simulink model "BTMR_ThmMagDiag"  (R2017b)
settings: Solver=FixedStepDiscrete  StartTime=0.0  StopTime=10  FixedStep=0.1  RelTol=1e-3  EnableMultiTasking=on
undefined symbols (not defined in the file or in its folder): bin2dec, BTMR_cntHtgCoolDiag_CW, BTMR_tAChrgHtgDiag_C, BTMR_tCoolDiag_CUR, BTMR_tDChrgHtgDiag_C, BTMR_tEnvTCool_CUR, BTMR_tHeatDiag_CUR, BTMR_tiThmCoolDebDiag_C, BTMR_tiThmCoolDiag_C, BTMR_tiThmCoolEndDiag_C, BTMR_tiThmHtgDebDiag_C, BTMR_tiThmHtgDiag_C, BTMR_tiThmHtgEndDiag_C, BTMR_tLowClntDiag_CUR, BTMR_tThmCoolLowLimt_C, enmThmDiagFlg
libraries: simulink x22

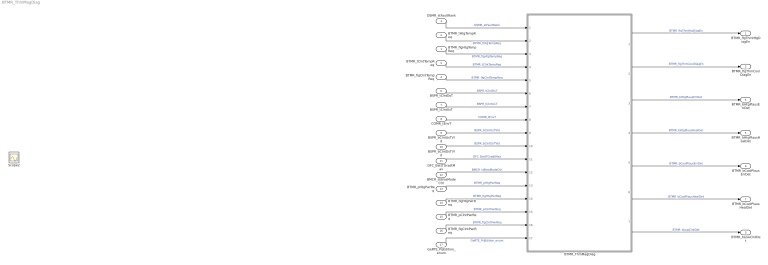
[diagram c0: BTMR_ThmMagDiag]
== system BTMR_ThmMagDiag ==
  BTMR_flgHtgTempReq : Inport
  BTMR_tHtgTempReq : Inport  Port=2
  DSMR_stFaultRank : Inport  Port=3
  BTMR_flgClntTempReq : Inport  Port=4
  BTMR_tClntTempReq : Inport  Port=5
  BSPR_tClntDsT : Inport  Port=6
  BSPR_tClntUsT : Inport  Port=7
  COMR_tEnvT : Inport  Port=8
  BSPR_bClntUsTVld : Inport  Port=9
  BSPR_bClntDsTVld : Inport  Port=10
  DFC_BattTGradtMax : Inport  Port=11
  BMCR_stBmsModeCtrl : Inport  Port=12
  BTMR_pHtgPwrReq : Inport  Port=13
  BTMR_flgHtgPwrReq : Inport  Port=14
  BTMR_pClntPwrReq : Inport  Port=15
  BTMR_flgClntPwrReq : Inport  Port=16
  GeRTE_PrjEdition_enum : Inport  Port=17
  BTMR_ThmMagDiag : Subsystem
  BTMR_flgThmHtgDiagEn : Outport
  BTMR_flgThmCoolDiagEn : Outport  Port=2
  BTMR_bLowClntDet : Outport  Port=3
  BTMR_bHtgPlausErrDet : Outport  Port=4
  BTMR_bHtgPlausHealDet : Outport  Port=5
  BTMR_bCoolPlausErrDet : Outport  Port=6
  BTMR_bCoolPlausHealDet : Outport  Port=7
  Scope2 : Scope
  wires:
  BTMR_tHtgTempReq/1 -> BTMR_ThmMagDiag/2(BTMR_tHtgTempReq)  "BTMR_tHtgTempReq"
  BTMR_flgHtgTempReq/1 -> BTMR_ThmMagDiag/3(BTMR_flgHtgTempReq)  "BTMR_flgHtgTempReq"
  BTMR_ThmMagDiag/1(BTMR_flgThmHtgDiagEn) -> BTMR_flgThmHtgDiagEn/1  "BTMR_flgThmHtgDiagEn"
  BTMR_ThmMagDiag/2(BTMR_flgThmCoolDiagEn) -> BTMR_flgThmCoolDiagEn/1  "BTMR_flgThmCoolDiagEn"
  BTMR_ThmMagDiag/4(BTMR_bHtgPlausHealDet) -> BTMR_bHtgPlausHealDet/1  "BTMR_bHtgPlausHealDet"
  BTMR_ThmMagDiag/3(BTMR_bHtgPlausErrDet) -> BTMR_bHtgPlausErrDet/1  "BTMR_bHtgPlausErrDet"
  BTMR_ThmMagDiag/5(BTMR_bCoolPlausErrDet) -> BTMR_bCoolPlausErrDet/1  "BTMR_bCoolPlausErrDet"
  BTMR_ThmMagDiag/6(BTMR_bCoolPlausHealDet) -> BTMR_bCoolPlausHealDet/1  "BTMR_bCoolPlausHealDet"
  BTMR_ThmMagDiag/7(BTMR_bLowClntDet) -> BTMR_bLowClntDet/1  "BTMR_bLowClntDet"
  DSMR_stFaultRank/1 -> BTMR_ThmMagDiag/1(DSMR_stFaultRank)  "DSMR_stFaultRank"
  BTMR_tClntTempReq/1 -> BTMR_ThmMagDiag/4(BTMR_tClntTempReq)  "BTMR_tClntTempReq"
  BTMR_flgClntTempReq/1 -> BTMR_ThmMagDiag/5(BTMR_flgClntTempReq)  "BTMR_flgClntTempReq"
  BSPR_tClntDsT/1 -> BTMR_ThmMagDiag/6(BSPR_tClntDsT)  "BSPR_tClntDsT"
  BSPR_tClntUsT/1 -> BTMR_ThmMagDiag/7(BSPR_tClntUsT)  "BSPR_tClntUsT"
  COMR_tEnvT/1 -> BTMR_ThmMagDiag/8(COMR_tEnvT)  "COMR_tEnvT"
  BSPR_bClntUsTVld/1 -> BTMR_ThmMagDiag/9(BSPR_bClntUsTVld)  "BSPR_bClntUsTVld"
  BSPR_bClntDsTVld/1 -> BTMR_ThmMagDiag/10(BSPR_bClntDsTVld)  "BSPR_bClntDsTVld"
  DFC_BattTGradtMax/1 -> BTMR_ThmMagDiag/11(DFC_BattTGradtMax)  "DFC_BattTGradtMax"
  BMCR_stBmsModeCtrl/1 -> BTMR_ThmMagDiag/12(BMCR_stBmsModeCtrl)  "BMCR_stBmsModeCtrl"
  BTMR_pHtgPwrReq/1 -> BTMR_ThmMagDiag/13(BTMR_pHtgPwrReq)  "BTMR_pHtgPwrReq"
  BTMR_flgHtgPwrReq/1 -> BTMR_ThmMagDiag/14(BTMR_flgHtgPwrReq)  "BTMR_flgHtgPwrReq"
  BTMR_flgClntPwrReq/1 -> BTMR_ThmMagDiag/16(BTMR_flgClntPwrReq)  "BTMR_flgClntPwrReq"
  BTMR_pClntPwrReq/1 -> BTMR_ThmMagDiag/15(BTMR_pClntPwrReq)  "BTMR_pClntPwrReq"
  GeRTE_PrjEdition_enum/1 -> BTMR_ThmMagDiag/17(GeRTE_PrjEdition_enum)  "GeRTE_PrjEdition_enum"

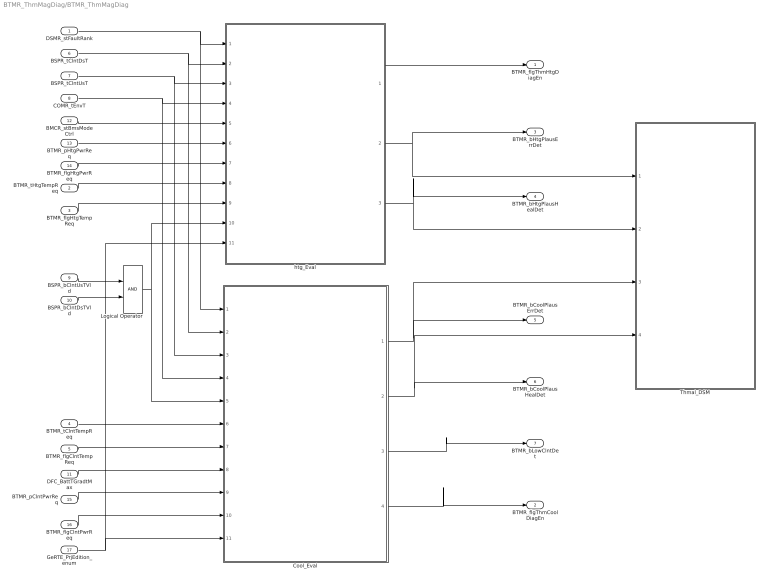
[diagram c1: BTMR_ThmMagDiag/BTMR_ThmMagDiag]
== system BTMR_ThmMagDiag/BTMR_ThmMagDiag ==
  DSMR_stFaultRank : Inport
  BTMR_tHtgTempReq : Inport  Port=2
  BTMR_flgHtgTempReq : Inport  Port=3
  BTMR_tClntTempReq : Inport  Port=4
  BTMR_flgClntTempReq : Inport  Port=5
  BSPR_tClntDsT : Inport  Port=6
  BSPR_tClntUsT : Inport  Port=7
  COMR_tEnvT : Inport  Port=8
  BSPR_bClntUsTVld : Inport  Port=9
  BSPR_bClntDsTVld : Inport  Port=10
  DFC_BattTGradtMax : Inport  Port=11  OutDataTypeStr=uint8
  BMCR_stBmsModeCtrl : Inport  Port=12
  BTMR_pHtgPwrReq : Inport  Port=13
  BTMR_flgHtgPwrReq : Inport  Port=14
  BTMR_pClntPwrReq : Inport  Port=15
  BTMR_flgClntPwrReq : Inport  Port=16
  GeRTE_PrjEdition_enum : Inport  Port=17
  Cool_Eval : Subsystem  TreatAsAtomicUnit=on
  Logical Operator : Logic  AllPortsSameDT=off  OutDataTypeStr=boolean
  Thmal_DSM : Subsystem
  htg_Eval : Subsystem  TreatAsAtomicUnit=on
  BTMR_flgThmHtgDiagEn : Outport
  BTMR_flgThmCoolDiagEn : Outport  Port=2
  BTMR_bHtgPlausErrDet : Outport  Port=3
  BTMR_bHtgPlausHealDet : Outport  Port=4
  BTMR_bCoolPlausErrDet : Outport  Port=5
  BTMR_bCoolPlausHealDet : Outport  Port=6
  BTMR_bLowClntDet : Outport  Port=7
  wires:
  DSMR_stFaultRank/1 -> Cool_Eval/1(DSMR_stFaultRank), htg_Eval/1(DSMR_stFaultRank)
  BSPR_tClntDsT/1 -> Cool_Eval/2(BSPR_tClntDsT), htg_Eval/2(BSPR_tClntDsT)
  BSPR_tClntUsT/1 -> Cool_Eval/3(BSPR_tClntUsT), htg_Eval/3(BSPR_tClntUsT)
  COMR_tEnvT/1 -> Cool_Eval/4(COMR_tEnvT), htg_Eval/4(COMR_tEnvT)
  htg_Eval/1(BTMR_flgThmHtgDiagEn) -> BTMR_flgThmHtgDiagEn/1
  BTMR_flgClntTempReq/1 -> Cool_Eval/7(BTMR_flgClntTempReq)
  BTMR_tClntTempReq/1 -> Cool_Eval/6(BTMR_tClntTempReq)
  BSPR_bClntUsTVld/1 -> Logical Operator/1
  BSPR_bClntDsTVld/1 -> Logical Operator/2
  Logical Operator/1 -> htg_Eval/10(BSPR_bClntTVld), Cool_Eval/5(BSPR_bClntTVld)
  Cool_Eval/3(BTMR_bLowClntDet) -> BTMR_bLowClntDet/1
  DFC_BattTGradtMax/1 -> Cool_Eval/8(DFC_BattTGradtMax)
  htg_Eval/2(BTMR_bHtgPlausErrDet) -> BTMR_bHtgPlausErrDet/1, Thmal_DSM/1(BTMR_bHtgPlausErrDet)
  htg_Eval/3(BTMR_bHtgPlausHealDet) -> BTMR_bHtgPlausHealDet/1, Thmal_DSM/2(BTMR_bHtgPlausHealDet)
  Cool_Eval/1(BTMR_bCoolPlausErrDet) -> Thmal_DSM/3(BTMR_bCoolPlausErrDet), BTMR_bCoolPlausErrDet/1
  Cool_Eval/2(BTMR_bCoolPlausHealDet) -> Thmal_DSM/4(BTMR_bCoolPlausHealDet), BTMR_bCoolPlausHealDet/1
  Cool_Eval/4(BTMR_flgThmCoolDiagEn) -> BTMR_flgThmCoolDiagEn/1
  BMCR_stBmsModeCtrl/1 -> htg_Eval/5(BMCR_stBmsModeCtrl)
  BTMR_pClntPwrReq/1 -> Cool_Eval/9(BTMR_pClntPwrReq)
  BTMR_flgClntPwrReq/1 -> Cool_Eval/10(BTMR_flgClntPwrReq)
  BTMR_pHtgPwrReq/1 -> htg_Eval/6(BTMR_pHtgPwrReq)
  BTMR_flgHtgPwrReq/1 -> htg_Eval/7(BTMR_flgHtgPwrReq)
  BTMR_flgHtgTempReq/1 -> htg_Eval/9(BTMR_flgHtgTempReq)
  BTMR_tHtgTempReq/1 -> htg_Eval/8(BTMR_tHtgTempReq)
  GeRTE_PrjEdition_enum/1 -> htg_Eval/11(GeRTE_PrjEdition_enum), Cool_Eval/11(GeRTE_PrjEdition_enum)

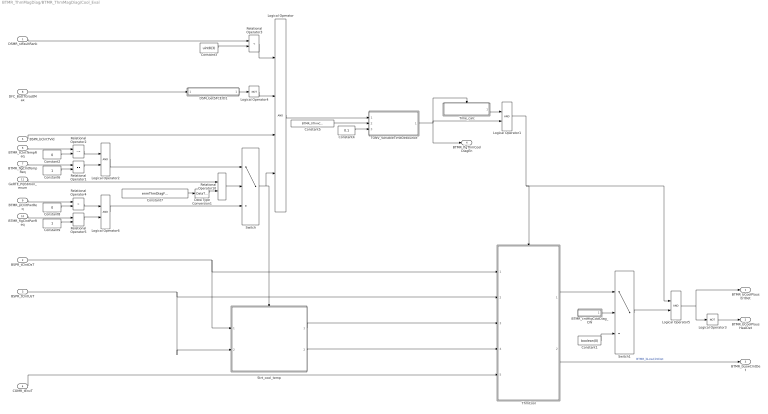
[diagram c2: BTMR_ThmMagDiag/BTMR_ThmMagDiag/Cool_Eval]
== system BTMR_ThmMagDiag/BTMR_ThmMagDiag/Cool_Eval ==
  DSMR_stFaultRank : Inport
  BSPR_tClntDsT : Inport  Port=2
  BSPR_tClntUsT : Inport  Port=3
  COMR_tEnvT : Inport  Port=4
  BSPR_bClntTVld : Inport  Port=5
  BTMR_tClntTempReq : Inport  Port=6
  BTMR_flgClntTempReq : Inport  Port=7
  DFC_BattTGradtMax : Inport  Port=8
  BTMR_pClntPwrReq : Inport  Port=9
  BTMR_flgClntPwrReq : Inport  Port=10
  GeRTE_PrjEdition_enum : Inport  Port=11
  BTMR_cntHtgCoolDiag_CW : Subsystem
  Constant1 : Constant  Value=boolean(0)
  Constant2 : Constant  Value=0  OutDataTypeStr=single
  Constant3 : Constant  Value=uint8(3)
  Constant4 : Constant  Value=0.1
  Constant5 : Constant  Value=BTMR_tiThmCoolDiag_C
  Constant6 : Constant  OutDataTypeStr=boolean
  Constant7 : Constant  Value=enmThmDiagFlg.TempReq  OutDataTypeStr=Enum: enmThmDiagFlg
  Constant8 : Constant  Value=0  OutDataTypeStr=single
  Constant9 : Constant  OutDataTypeStr=boolean
  DSM_GetSFCErD1 : Subsystem  TreatAsAtomicUnit=on  RTWFcnName=TONV_10msTimeDebounce  RTWFileName=SrvLib
  Data Type Conversion1 : DataTypeConversion  OutDataTypeStr=uint8
  Logical Operator : Logic  Inputs=4  AllPortsSameDT=off  OutDataTypeStr=boolean
  Logical Operator{1..2,5..6} (4 alike) : Logic  AllPortsSameDT=off  OutDataTypeStr=boolean
  Logical Operator3 : Logic  Operator=NOT  Inputs=1  AllPortsSameDT=off  OutDataTypeStr=boolean
  Logical Operator4 : Logic  Operator=NOT  Inputs=1  AllPortsSameDT=off  OutDataTypeStr=boolean
  Relational Operator1 : RelationalOperator  Operator===  OutDataTypeStr=boolean  RndMeth=Simplest
  Relational Operator10 : RelationalOperator  Operator===  OutDataTypeStr=boolean  RndMeth=Simplest
  Relational Operator2 : RelationalOperator  Operator=~=  OutDataTypeStr=boolean  RndMeth=Simplest
  Relational Operator3 : RelationalOperator  Operator=<  OutDataTypeStr=boolean  RndMeth=Simplest
  Relational Operator4 : RelationalOperator  Operator=>  OutDataTypeStr=boolean  RndMeth=Simplest
  Relational Operator5 : RelationalOperator  Operator===  OutDataTypeStr=boolean  RndMeth=Simplest
  Strt_cool_temp : Subsystem  TreatAsAtomicUnit=on
  Switch : Switch  Criteria=u2 > Threshold
  Switch1 : Switch  Criteria=u2 > Threshold
  TONV_VariableTimeDebounce : Subsystem  TreatAsAtomicUnit=on  RTWFcnName=TONV_VariableTimeDebounce  RTWFileName=SrvLib
  ThmCool : Subsystem  TreatAsAtomicUnit=on
  Time_calc : Subsystem  TreatAsAtomicUnit=on
  BTMR_bCoolPlausErrDet : Outport
  BTMR_bCoolPlausHealDet : Outport  Port=2
  BTMR_bLowClntDet : Outport  Port=3
  BTMR_flgThmCoolDiagEn : Outport  Port=4
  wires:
  Constant2/1 -> Relational Operator2/2
  Constant3/1 -> Relational Operator3/2
  Constant4/1 -> TONV_VariableTimeDebounce/3(dT)
  Constant5/1 -> TONV_VariableTimeDebounce/2(T)
  Relational Operator2/1 -> Logical Operator2/1
  Relational Operator3/1 -> Logical Operator/1
  BSPR_tClntDsT/1 -> ThmCool/1(BSPR_tClntDsT), Strt_cool_temp/1(BSPR_tClntDsT)
  BSPR_tClntUsT/1 -> ThmCool/2(BSPR_tClntUsT), Strt_cool_temp/2(BSPR_tClntUsT)
  DSMR_stFaultRank/1 -> Relational Operator3/1
  BTMR_tClntTempReq/1 -> Relational Operator2/1
  TONV_VariableTimeDebounce/1(y) -> Logical Operator1/2, BTMR_flgThmCoolDiagEn/1, Time_calc/Enable
  Time_calc/1(BTMR_flgThmCoolTimeEn) -> Logical Operator1/1
  Logical Operator1/1 -> Logical Operator5/1, ThmCool/Enable
  Constant1/1 -> Switch1/3
  ThmCool/1(BTMR_bCoolPlausErrDet) -> Switch1/1
  Logical Operator3/1 -> BTMR_bCoolPlausHealDet/1
  BTMR_cntHtgCoolDiag_CW/1(CW) -> Switch1/2
  Switch/1 -> Strt_cool_temp/Trigger, Logical Operator/4
  BSPR_bClntTVld/1 -> Logical Operator/3
  ThmCool/2(BTMR_bLowClntDet) -> BTMR_bLowClntDet/1  "BTMR_bLowClntDet"
  Strt_cool_temp/1(BSPR_tClntDsStrtCool) -> ThmCool/3(BSPR_tClntDsStrtCool)
  Strt_cool_temp/2(BSPR_tClntUsStrtCool) -> ThmCool/4(BSPR_tClntUsStrtCool)
  COMR_tEnvT/1 -> ThmCool/5(COMR_tEnvT)
  Logical Operator4/1 -> Logical Operator/2
  DFC_BattTGradtMax/1 -> DSM_GetSFCErD1/1(DFC)
  DSM_GetSFCErD1/1(y) -> Logical Operator4/1
  Logical Operator/1 -> TONV_VariableTimeDebounce/1(u)
  Switch1/1 -> Logical Operator5/2
  Logical Operator5/1 -> BTMR_bCoolPlausErrDet/1, Logical Operator3/1
  Constant6/1 -> Relational Operator1/2
  BTMR_flgClntTempReq/1 -> Relational Operator1/1
  Relational Operator1/1 -> Logical Operator2/2
  Relational Operator10/1 -> Switch/2
  Relational Operator4/1 -> Logical Operator6/1
  Constant8/1 -> Relational Operator4/2
  BTMR_pClntPwrReq/1 -> Relational Operator4/1
  Logical Operator2/1 -> Switch/1
  Logical Operator6/1 -> Switch/3
  BTMR_flgClntPwrReq/1 -> Relational Operator5/1
  Constant9/1 -> Relational Operator5/2
  Relational Operator5/1 -> Logical Operator6/2
  Data Type Conversion1/1 -> Relational Operator10/2
  GeRTE_PrjEdition_enum/1 -> Relational Operator10/1
  Constant7/1 -> Data Type Conversion1/1

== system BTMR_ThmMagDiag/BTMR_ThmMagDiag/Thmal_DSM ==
  BTMR_bHtgPlausErrDet : Inport
  BTMR_bHtgPlausHealDet : Inport  Port=2
  BTMR_bCoolPlausErrDet : Inport  Port=3
  BTMR_bCoolPlausHealDet : Inport  Port=4
  DSM_ReportCheck2 : Subsystem  TreatAsAtomicUnit=on  RTWFcnName=DSM_ReportCheck  RTWFileName=SrvLib
  DSM_ReportCheck3 : Subsystem  TreatAsAtomicUnit=on  RTWFcnName=DSM_ReportCheck  RTWFileName=SrvLib
  Data Store Read : DataStoreRead  DataStoreName=DFC_HtgPerfPlaus
  Data Store Read1 : DataStoreRead  DataStoreName=DFC_CoolPerfPlaus
  Data Store Write : DataStoreWrite  DataStoreName=DFC_HtgPerfPlaus
  Data Store Write1 : DataStoreWrite  DataStoreName=DFC_CoolPerfPlaus
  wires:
  DSM_ReportCheck2/1(Dfc_id) -> Data Store Write1/1
  Data Store Read1/1 -> DSM_ReportCheck2/1(Dfc_id_nv)
  Data Store Read/1 -> DSM_ReportCheck3/1(Dfc_id_nv)
  DSM_ReportCheck3/1(Dfc_id) -> Data Store Write/1
  BTMR_bHtgPlausErrDet/1 -> DSM_ReportCheck3/2(Err)
  BTMR_bHtgPlausHealDet/1 -> DSM_ReportCheck3/3(Heal)
  BTMR_bCoolPlausErrDet/1 -> DSM_ReportCheck2/2(Err)
  BTMR_bCoolPlausHealDet/1 -> DSM_ReportCheck2/3(Heal)

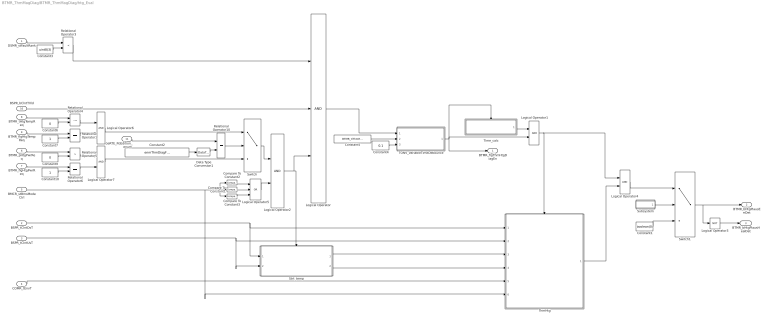
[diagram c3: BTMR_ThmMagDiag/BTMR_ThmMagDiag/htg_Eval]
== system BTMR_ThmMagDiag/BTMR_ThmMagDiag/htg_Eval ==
  DSMR_stFaultRank : Inport
  BSPR_tClntDsT : Inport  Port=2
  BSPR_tClntUsT : Inport  Port=3
  COMR_tEnvT : Inport  Port=4
  BMCR_stBmsModeCtrl : Inport  Port=5
  BTMR_pHtgPwrReq : Inport  Port=6
  BTMR_flgHtgPwrReq : Inport  Port=7
  BTMR_tHtgTempReq : Inport  Port=8
  BTMR_flgHtgTempReq : Inport  Port=9
  BSPR_bClntTVld : Inport  Port=10
  GeRTE_PrjEdition_enum : Inport  Port=11
  Compare To Constant1 : simulink/Logic and Bit Operations/Compare To Constant  relop===  const=5  OutDataTypeStr=boolean
  Compare To Constant2 : simulink/Logic and Bit Operations/Compare To Constant  relop===  const=6  OutDataTypeStr=boolean
  Compare To Constant3 : simulink/Logic and Bit Operations/Compare To Constant  relop===  const=11  OutDataTypeStr=boolean
  Constant1 : Constant  Value=boolean(0)
  Constant10 : Constant  OutDataTypeStr=boolean
  Constant2 : Constant  Value=enmThmDiagFlg.TempReq  OutDataTypeStr=Enum: enmThmDiagFlg
  Constant3 : Constant  Value=uint8(3)
  Constant4 : Constant  Value=0.1
  Constant5 : Constant  Value=BTMR_tiThmHtgDiag_C
  Constant6 : Constant  Value=0  OutDataTypeStr=single
  Constant7 : Constant  OutDataTypeStr=boolean
  Constant9 : Constant  Value=0  OutDataTypeStr=single
  Data Type Conversion1 : DataTypeConversion  OutDataTypeStr=uint8
  Logical Operator : Logic  Inputs=3  AllPortsSameDT=off  OutDataTypeStr=boolean
  Logical Operator{1..2,4,6..7} (5 alike) : Logic  AllPortsSameDT=off  OutDataTypeStr=boolean
  Logical Operator3 : Logic  Operator=NOT  Inputs=1  AllPortsSameDT=off  OutDataTypeStr=boolean
  Logical Operator5 : Logic  Operator=OR  Inputs=3  AllPortsSameDT=off  OutDataTypeStr=boolean
  Relational Operator1 : RelationalOperator  Operator===  OutDataTypeStr=boolean  RndMeth=Simplest
  Relational Operator10 : RelationalOperator  Operator===  OutDataTypeStr=boolean  RndMeth=Simplest
  Relational Operator3 : RelationalOperator  Operator=<  OutDataTypeStr=boolean  RndMeth=Simplest
  Relational Operator4 : RelationalOperator  Operator=~=  OutDataTypeStr=boolean  RndMeth=Simplest
  Relational Operator5 : RelationalOperator  Operator=>  OutDataTypeStr=boolean  RndMeth=Simplest
  Relational Operator6 : RelationalOperator  Operator===  OutDataTypeStr=boolean  RndMeth=Simplest
  Strt_temp : Subsystem  TreatAsAtomicUnit=on
  Subsystem : Subsystem
  Switch : Switch  Criteria=u2 > Threshold
  Switch1 : Switch  Criteria=u2 > Threshold
  TONV_VariableTimeDebounce : Subsystem  TreatAsAtomicUnit=on  RTWFcnName=TONV_VariableTimeDebounce  RTWFileName=SrvLib
  ThmHtg : Subsystem  TreatAsAtomicUnit=on
  Time_calc : Subsystem  TreatAsAtomicUnit=on
  BTMR_flgThmHtgDiagEn : Outport
  BTMR_bHtgPlausErrDet : Outport  Port=2
  BTMR_bHtgPlausHealDet : Outport  Port=3
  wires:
  DSMR_stFaultRank/1 -> Relational Operator3/1
  Constant3/1 -> Relational Operator3/2
  Logical Operator/1 -> TONV_VariableTimeDebounce/1(u)
  Constant4/1 -> TONV_VariableTimeDebounce/3(dT)
  Constant5/1 -> TONV_VariableTimeDebounce/2(T)
  TONV_VariableTimeDebounce/1(y) -> Logical Operator1/2, BTMR_flgThmHtgDiagEn/1, Time_calc/Enable
  COMR_tEnvT/1 -> ThmHtg/5(COMR_tEnvT)
  BSPR_tClntDsT/1 -> Strt_temp/1(BSPR_tClntDsT), ThmHtg/1(BSPR_tClntDsT)
  BSPR_tClntUsT/1 -> Strt_temp/2(BSPR_tClntUsT), ThmHtg/2(BSPR_tClntUsT)
  Strt_temp/2(BSPR_tClntUsStrtHtg) -> ThmHtg/4(BSPR_tClntUsStrtHtg)
  Strt_temp/1(BSPR_tClntDsStrtHtg) -> ThmHtg/3(BSPR_tClntDsStrtHtg)
  Relational Operator3/1 -> Logical Operator/1
  Time_calc/1(BTMR_flgThmHtgTimeEn) -> Logical Operator1/1
  Logical Operator1/1 -> ThmHtg/Enable, Logical Operator4/1
  Constant1/1 -> Switch1/3
  Switch1/1 -> Logical Operator3/1, BTMR_bHtgPlausErrDet/1
  Logical Operator3/1 -> BTMR_bHtgPlausHealDet/1
  Subsystem/1(CW) -> Switch1/2
  ThmHtg/1(BTMR_bHtgPlausErrDet) -> Logical Operator4/2
  Logical Operator4/1 -> Switch1/1
  BMCR_stBmsModeCtrl/1 -> ThmHtg/6(BMCR_stBmsModeCtrl), Compare To Constant3/1, Compare To Constant2/1, Compare To Constant1/1
  Logical Operator2/1 -> Strt_temp/Trigger, Logical Operator/3
  Compare To Constant2/1 -> Logical Operator5/1
  Compare To Constant1/1 -> Logical Operator5/2
  Logical Operator5/1 -> Logical Operator2/2
  Compare To Constant3/1 -> Logical Operator5/3
  Logical Operator7/1 -> Switch/3
  Relational Operator10/1 -> Switch/2
  Relational Operator4/1 -> Logical Operator6/1
  Relational Operator1/1 -> Logical Operator6/2
  Constant7/1 -> Relational Operator1/2
  Constant9/1 -> Relational Operator5/2
  BTMR_flgHtgTempReq/1 -> Relational Operator1/1
  Relational Operator5/1 -> Logical Operator7/1
  Logical Operator6/1 -> Switch/1
  Relational Operator6/1 -> Logical Operator7/2
  Constant10/1 -> Relational Operator6/2
  Constant6/1 -> Relational Operator4/2
  BTMR_tHtgTempReq/1 -> Relational Operator4/1
  BTMR_pHtgPwrReq/1 -> Relational Operator5/1
  BTMR_flgHtgPwrReq/1 -> Relational Operator6/1
  Switch/1 -> Logical Operator2/1
  BSPR_bClntTVld/1 -> Logical Operator/2
  Data Type Conversion1/1 -> Relational Operator10/2
  GeRTE_PrjEdition_enum/1 -> Relational Operator10/1
  Constant2/1 -> Data Type Conversion1/1

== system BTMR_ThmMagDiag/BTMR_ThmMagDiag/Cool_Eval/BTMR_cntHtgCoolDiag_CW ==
  Bitwise Operator : simulink/Logic and Bit Operations/Bitwise Operator  logicop=AND  UseBitMask=on  BitMask=bin2dec('00000010')  BitMaskRealWorld=Stored Integer
  Compare To Constant1 : simulink/Logic and Bit Operations/Compare To Constant  relop===  const=2  OutDataTypeStr=boolean
  Constant7 : Constant  Value=BTMR_cntHtgCoolDiag_CW
  CW : Outport
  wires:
  Compare To Constant1/1 -> CW/1
  Constant7/1 -> Bitwise Operator/1
  Bitwise Operator/1 -> Compare To Constant1/1

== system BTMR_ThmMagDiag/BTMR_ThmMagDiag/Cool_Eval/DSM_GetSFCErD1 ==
  DFC : Inport  OutDataTypeStr=uint8
  DFC_IsoChkLv1_1 : simulink/Logic and Bit Operations/Bitwise Operator  logicop=AND  UseBitMask=on  BitMask=bin2dec('00010000')  BitMaskRealWorld=Stored Integer
  DFC_IsoChkLv1_1_compare : simulink/Logic and Bit Operations/Compare To Constant  relop===  const=16  OutDataTypeStr=boolean
  y : Outport
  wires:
  DFC_IsoChkLv1_1/1 -> DFC_IsoChkLv1_1_compare/1
  DFC/1 -> DFC_IsoChkLv1_1/1
  DFC_IsoChkLv1_1_compare/1 -> y/1

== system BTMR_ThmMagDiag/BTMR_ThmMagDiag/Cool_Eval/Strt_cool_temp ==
  BSPR_tClntDsT : Inport
  BSPR_tClntUsT : Inport  Port=2
  Trigger : TriggerPort  VariantControl=Variant
  BSPR_tClntDsStrtCool : Outport
  BSPR_tClntUsStrtCool : Outport  Port=2
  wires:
  BSPR_tClntDsT/1 -> BSPR_tClntDsStrtCool/1  "BSPR_tClntDsStrtCool"
  BSPR_tClntUsT/1 -> BSPR_tClntUsStrtCool/1  "BSPR_tClntUsStrtCool"

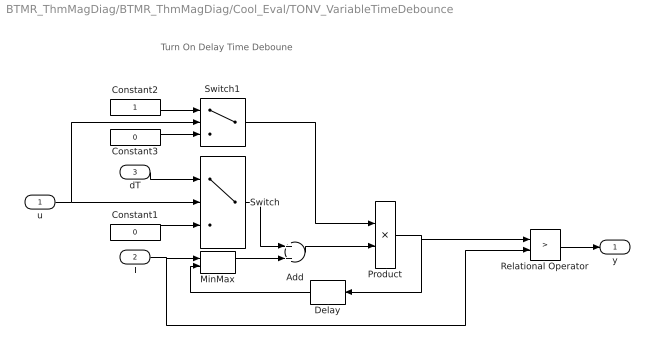
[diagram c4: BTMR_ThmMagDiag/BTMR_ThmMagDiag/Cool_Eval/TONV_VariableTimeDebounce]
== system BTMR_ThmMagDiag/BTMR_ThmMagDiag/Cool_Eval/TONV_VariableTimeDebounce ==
  note: Turn On Delay Time Deboune
  u : Inport
  T : Inport  Port=2
  dT : Inport  Port=3
  Add : Sum
  Constant1 : Constant  Value=0  OutDataTypeStr=single
  Constant2 : Constant  OutDataTypeStr=uint8
  Constant3 : Constant  Value=0  OutDataTypeStr=uint8
  Delay : Delay  DelayLength=1  InitialCondition=0
  MinMax : MinMax  Inputs=2
  Product : Product  OutMin=[0]  OutMax=[65535]  OutDataTypeStr=single
  Relational Operator : RelationalOperator  Operator=>  OutDataTypeStr=boolean  RndMeth=Simplest
  Switch : Switch  Criteria=u2 ~= 0
  Switch1 : Switch  Criteria=u2 ~= 0
  y : Outport
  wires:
  Switch1/1 -> Product/1
  Constant3/1 -> Switch1/3
  Constant2/1 -> Switch1/1
  u/1 -> Switch1/2, Switch/2
  dT/1 -> Switch/1
  Constant1/1 -> Switch/3
  Add/1 -> Product/2
  Product/1 -> Relational Operator/1, Delay/1
  Switch/1 -> Add/1
  Delay/1 -> MinMax/2
  Relational Operator/1 -> y/1
  T/1 -> MinMax/1, Relational Operator/2
  MinMax/1 -> Add/2

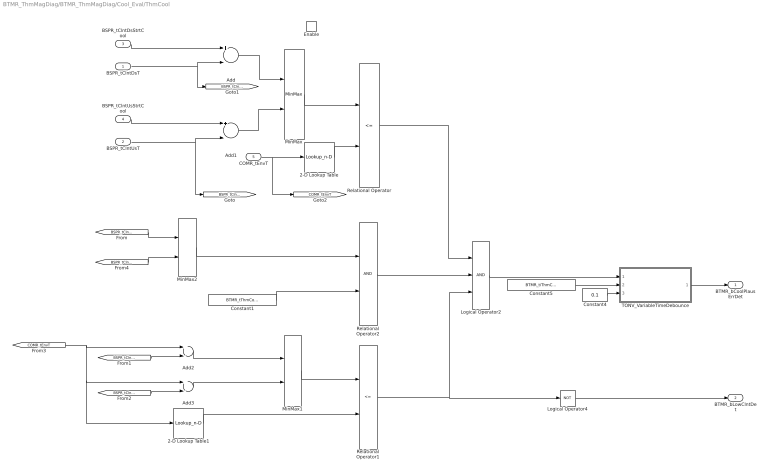
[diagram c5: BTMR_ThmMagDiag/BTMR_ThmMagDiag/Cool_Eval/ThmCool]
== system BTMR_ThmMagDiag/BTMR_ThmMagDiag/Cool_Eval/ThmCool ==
  BSPR_tClntDsT : Inport
  BSPR_tClntUsT : Inport  Port=2
  BSPR_tClntDsStrtCool : Inport  Port=3
  BSPR_tClntUsStrtCool : Inport  Port=4
  COMR_tEnvT : Inport  Port=5
  Enable : EnablePort  StatesWhenEnabling=reset
  2-D Lookup Table : Lookup_n-D  NumberOfTableDimensions=1  BreakpointsForDimension1=BTMR_tEnvTCool_CUR  BreakpointsForDimension2=[1:3]  Table=BTMR_tCoolDiag_CUR  InternalRulePriority=Speed  RndMeth=Simplest
  2-D Lookup Table1 : Lookup_n-D  NumberOfTableDimensions=1  BreakpointsForDimension1=BTMR_tEnvTCool_CUR  BreakpointsForDimension2=[1:3]  Table=BTMR_tLowClntDiag_CUR  InternalRulePriority=Speed  RndMeth=Simplest
  Add{,1..3} (4 alike) : Sum  Inputs=+-
  Constant1 : Constant  Value=BTMR_tThmCoolLowLimt_C
  Constant4 : Constant  Value=0.1
  Constant5 : Constant  Value=BTMR_tiThmCoolDebDiag_C
  Logical Operator2 : Logic  Inputs=3  OutDataTypeStr=boolean
  Logical Operator4 : Logic  Operator=NOT  Inputs=1  AllPortsSameDT=off  OutDataTypeStr=boolean
  MinMax : MinMax  Function=max  Inputs=2
  MinMax1 : MinMax  Function=max  Inputs=2
  MinMax2 : MinMax  Inputs=2
  Relational Operator : RelationalOperator  Operator=<=  OutDataTypeStr=boolean  RndMeth=Simplest
  Relational Operator1 : RelationalOperator  Operator=<=  OutDataTypeStr=boolean  RndMeth=Simplest
  Relational Operator2 : RelationalOperator  OutDataTypeStr=boolean  RndMeth=Simplest
  TONV_VariableTimeDebounce : Subsystem  TreatAsAtomicUnit=on  RTWFcnName=TONV_VariableTimeDebounce  RTWFileName=SrvLib
  BTMR_bCoolPlausErrDet : Outport
  BTMR_bLowClntDet : Outport  Port=2
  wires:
  Add/1 -> MinMax/1
  Add1/1 -> MinMax/2
  MinMax/1 -> Relational Operator/1
  COMR_tEnvT/1 -> 2-D Lookup Table/1, [COMR_tEnvT]
  2-D Lookup Table/1 -> Relational Operator/2
  BSPR_tClntDsStrtCool/1 -> Add/1
  Constant4/1 -> TONV_VariableTimeDebounce/3(dT)
  Constant5/1 -> TONV_VariableTimeDebounce/2(T)
  TONV_VariableTimeDebounce/1(y) -> BTMR_bCoolPlausErrDet/1
  BSPR_tClntDsT/1 -> Add/2, [BSPR_tClntDsT]
  Relational Operator/1 -> Logical Operator2/1
  Logical Operator2/1 -> TONV_VariableTimeDebounce/1(u)
  Add2/1 -> MinMax1/1
  Add3/1 -> MinMax1/2
  MinMax1/1 -> Relational Operator1/1
  2-D Lookup Table1/1 -> Relational Operator1/2
  Relational Operator1/1 -> Logical Operator4/1, Logical Operator2/3
  [COMR_tEnvT] -> Add2/1, Add3/1, 2-D Lookup Table1/1
  [BSPR_tClntUsT] -> Add3/2
  [BSPR_tClntDsT] -> Add2/2
  BSPR_tClntUsStrtCool/1 -> Add1/1
  BSPR_tClntUsT/1 -> [BSPR_tClntUsT], Add1/2
  Logical Operator4/1 -> BTMR_bLowClntDet/1
  [BSPR_tClntDsT] -> MinMax2/1
  [BSPR_tClntUsT] -> MinMax2/2
  MinMax2/1 -> Relational Operator2/1
  Relational Operator2/1 -> Logical Operator2/2
  Constant1/1 -> Relational Operator2/2

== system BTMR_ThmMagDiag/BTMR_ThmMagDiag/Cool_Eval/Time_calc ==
  Enable : EnablePort  StatesWhenEnabling=reset
  Add1 : Sum
  Constant : Constant  Value=0.1  OutDataTypeStr=uint8
  Constant5 : Constant  Value=BTMR_tiThmCoolEndDiag_C
  Delay1 : Delay  DelayLength=1  InitialCondition=0
  Logical Operator : Logic  Operator=NOT  Inputs=1  AllPortsSameDT=off  OutDataTypeStr=boolean
  Relational Operator : RelationalOperator  Operator=>  OutDataTypeStr=boolean  RndMeth=Simplest
  BTMR_flgThmCoolTimeEn : Outport
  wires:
  Constant5/1 -> Relational Operator/2
  Relational Operator/1 -> Logical Operator/1
  Logical Operator/1 -> BTMR_flgThmCoolTimeEn/1  "BTMR_flgThmCoolTimeEn"
  Constant/1 -> Add1/1
  Delay1/1 -> Add1/2
  Add1/1 -> Delay1/1, Relational Operator/1

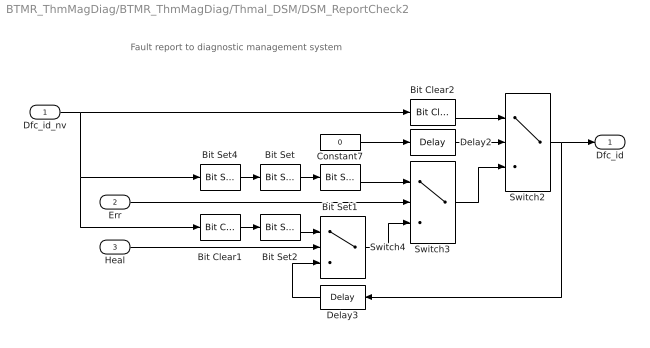
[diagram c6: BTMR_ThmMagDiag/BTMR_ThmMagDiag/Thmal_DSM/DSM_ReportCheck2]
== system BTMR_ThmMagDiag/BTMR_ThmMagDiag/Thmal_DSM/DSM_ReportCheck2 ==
  note: Fault report to diagnostic management system
  Dfc_id_nv : Inport  OutDataTypeStr=uint8
  Err : Inport  Port=2
  Heal : Inport  Port=3
  Bit Clear1 : simulink/Logic and Bit Operations/Bit Clear  iBit=4
  Bit Clear2 : simulink/Logic and Bit Operations/Bit Clear  iBit=3
  Bit Set : simulink/Logic and Bit Operations/Bit Set  iBit=4
  Bit Set1 : simulink/Logic and Bit Operations/Bit Set  iBit=3
  Bit Set2 : simulink/Logic and Bit Operations/Bit Set  iBit=3
  Bit Set4 : simulink/Logic and Bit Operations/Bit Set  iBit=7
  Constant7 : Constant  Value=0  OutDataTypeStr=boolean
  Delay2 : Delay  DelayLength=1  InitialCondition=1
  Delay3 : Delay  DelayLength=1  InitialCondition=0
  Switch2 : Switch  Criteria=u2 ~= 0
  Switch3 : Switch  Criteria=u2 ~= 0
  Switch4 : Switch  Criteria=u2 ~= 0
  Dfc_id : Outport  OutDataTypeStr=uint8
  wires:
  Dfc_id_nv/1 -> Bit Clear2/1, Bit Set4/1, Bit Clear1/1
  Bit Set4/1 -> Bit Set/1
  Constant7/1 -> Delay2/1
  Delay2/1 -> Switch2/2
  Switch3/1 -> Switch2/3
  Bit Clear2/1 -> Switch2/1
  Switch2/1 -> Delay3/1, Dfc_id/1
  Bit Set1/1 -> Switch3/1
  Bit Set/1 -> Bit Set1/1
  Switch4/1 -> Switch3/3
  Err/1 -> Switch3/2
  Bit Set2/1 -> Switch4/1
  Bit Clear1/1 -> Bit Set2/1
  Delay3/1 -> Switch4/3
  Heal/1 -> Switch4/2

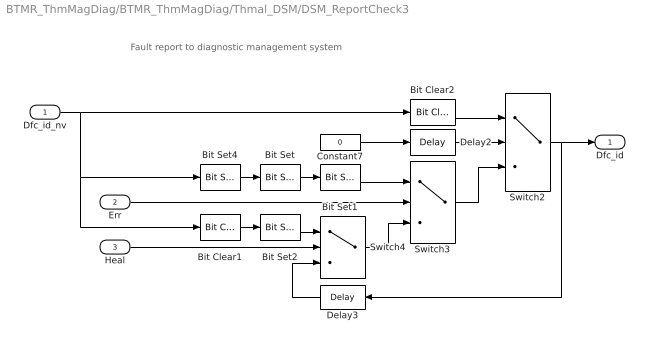
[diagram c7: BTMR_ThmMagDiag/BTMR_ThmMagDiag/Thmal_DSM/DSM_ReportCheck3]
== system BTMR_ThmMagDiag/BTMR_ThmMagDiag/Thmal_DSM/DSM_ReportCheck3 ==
  note: Fault report to diagnostic management system
  Dfc_id_nv : Inport  OutDataTypeStr=uint8
  Err : Inport  Port=2
  Heal : Inport  Port=3
  Bit Clear1 : simulink/Logic and Bit Operations/Bit Clear  iBit=4
  Bit Clear2 : simulink/Logic and Bit Operations/Bit Clear  iBit=3
  Bit Set : simulink/Logic and Bit Operations/Bit Set  iBit=4
  Bit Set1 : simulink/Logic and Bit Operations/Bit Set  iBit=3
  Bit Set2 : simulink/Logic and Bit Operations/Bit Set  iBit=3
  Bit Set4 : simulink/Logic and Bit Operations/Bit Set  iBit=7
  Constant7 : Constant  Value=0  OutDataTypeStr=boolean
  Delay2 : Delay  DelayLength=1  InitialCondition=1
  Delay3 : Delay  DelayLength=1  InitialCondition=0
  Switch2 : Switch  Criteria=u2 ~= 0
  Switch3 : Switch  Criteria=u2 ~= 0
  Switch4 : Switch  Criteria=u2 ~= 0
  Dfc_id : Outport  OutDataTypeStr=uint8
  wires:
  Heal/1 -> Switch4/2
  Delay3/1 -> Switch4/3
  Bit Clear1/1 -> Bit Set2/1
  Bit Set2/1 -> Switch4/1
  Err/1 -> Switch3/2
  Switch4/1 -> Switch3/3
  Bit Set/1 -> Bit Set1/1
  Bit Set1/1 -> Switch3/1
  Switch2/1 -> Dfc_id/1, Delay3/1
  Bit Clear2/1 -> Switch2/1
  Switch3/1 -> Switch2/3
  Delay2/1 -> Switch2/2
  Constant7/1 -> Delay2/1
  Bit Set4/1 -> Bit Set/1
  Dfc_id_nv/1 -> Bit Clear1/1, Bit Set4/1, Bit Clear2/1

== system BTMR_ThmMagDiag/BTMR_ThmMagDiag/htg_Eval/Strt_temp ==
  BSPR_tClntDsT : Inport
  BSPR_tClntUsT : Inport  Port=2
  Trigger : TriggerPort  VariantControl=Variant
  BSPR_tClntDsStrtHtg : Outport
  BSPR_tClntUsStrtHtg : Outport  Port=2
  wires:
  BSPR_tClntDsT/1 -> BSPR_tClntDsStrtHtg/1  "BSPR_tClntDsStrtHtg"
  BSPR_tClntUsT/1 -> BSPR_tClntUsStrtHtg/1  "BSPR_tClntUsStrtHtg"

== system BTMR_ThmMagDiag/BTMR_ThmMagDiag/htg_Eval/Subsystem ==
  Bitwise Operator : simulink/Logic and Bit Operations/Bitwise Operator  logicop=AND  UseBitMask=on  BitMask=bin2dec('00000001')  BitMaskRealWorld=Stored Integer
  Compare To Constant1 : simulink/Logic and Bit Operations/Compare To Constant  relop===  const=1  OutDataTypeStr=boolean
  Constant7 : Constant  Value=BTMR_cntHtgCoolDiag_CW
  CW : Outport
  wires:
  Compare To Constant1/1 -> CW/1
  Bitwise Operator/1 -> Compare To Constant1/1
  Constant7/1 -> Bitwise Operator/1

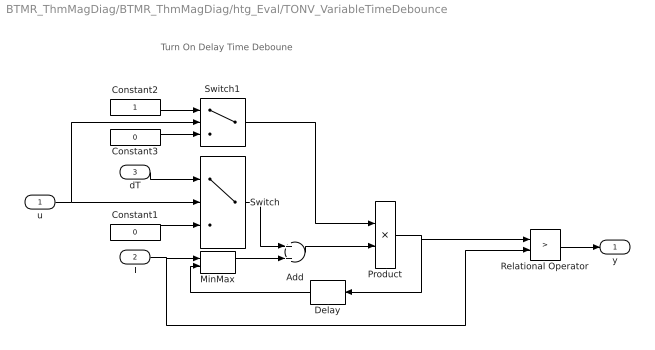
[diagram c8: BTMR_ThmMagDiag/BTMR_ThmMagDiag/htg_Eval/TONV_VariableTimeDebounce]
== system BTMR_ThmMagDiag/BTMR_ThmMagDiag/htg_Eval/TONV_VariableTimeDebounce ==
  note: Turn On Delay Time Deboune
  u : Inport
  T : Inport  Port=2
  dT : Inport  Port=3
  Add : Sum
  Constant1 : Constant  Value=0  OutDataTypeStr=single
  Constant2 : Constant  OutDataTypeStr=uint8
  Constant3 : Constant  Value=0  OutDataTypeStr=uint8
  Delay : Delay  DelayLength=1  InitialCondition=0
  MinMax : MinMax  Inputs=2
  Product : Product  OutMin=[0]  OutMax=[65535]  OutDataTypeStr=single
  Relational Operator : RelationalOperator  Operator=>  OutDataTypeStr=boolean  RndMeth=Simplest
  Switch : Switch  Criteria=u2 ~= 0
  Switch1 : Switch  Criteria=u2 ~= 0
  y : Outport
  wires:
  Switch1/1 -> Product/1
  Constant3/1 -> Switch1/3
  Constant2/1 -> Switch1/1
  u/1 -> Switch1/2, Switch/2
  dT/1 -> Switch/1
  Constant1/1 -> Switch/3
  Add/1 -> Product/2
  Product/1 -> Relational Operator/1, Delay/1
  Switch/1 -> Add/1
  Delay/1 -> MinMax/2
  Relational Operator/1 -> y/1
  T/1 -> MinMax/1, Relational Operator/2
  MinMax/1 -> Add/2

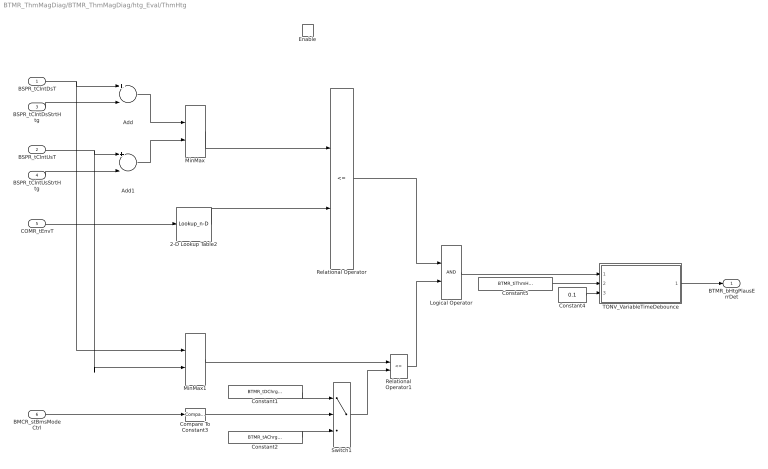
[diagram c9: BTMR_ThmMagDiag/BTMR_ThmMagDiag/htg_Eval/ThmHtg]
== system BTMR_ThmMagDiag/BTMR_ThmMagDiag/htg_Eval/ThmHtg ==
  BSPR_tClntDsT : Inport
  BSPR_tClntUsT : Inport  Port=2
  BSPR_tClntDsStrtHtg : Inport  Port=3
  BSPR_tClntUsStrtHtg : Inport  Port=4
  COMR_tEnvT : Inport  Port=5
  BMCR_stBmsModeCtrl : Inport  Port=6
  Enable : EnablePort  StatesWhenEnabling=reset
  2-D Lookup Table2 : Lookup_n-D  NumberOfTableDimensions=1  BreakpointsForDimension1=BTMR_tEnvTCool_CUR  BreakpointsForDimension2=[1:3]  Table=BTMR_tHeatDiag_CUR  InternalRulePriority=Speed  RndMeth=Simplest
  Add : Sum  Inputs=+-
  Add1 : Sum  Inputs=+-
  Compare To Constant3 : simulink/Logic and Bit Operations/Compare To Constant  relop===  const=5  OutDataTypeStr=boolean
  Constant1 : Constant  Value=BTMR_tDChrgHtgDiag_C
  Constant2 : Constant  Value=BTMR_tAChrgHtgDiag_C
  Constant4 : Constant  Value=0.1
  Constant5 : Constant  Value=BTMR_tiThmHtgDebDiag_C
  Logical Operator : Logic  AllPortsSameDT=off  OutDataTypeStr=boolean
  MinMax : MinMax  Function=max  Inputs=2
  MinMax1 : MinMax  Inputs=2
  Relational Operator : RelationalOperator  Operator=<=  OutDataTypeStr=boolean  RndMeth=Simplest
  Relational Operator1 : RelationalOperator  Operator=<=  OutDataTypeStr=boolean  RndMeth=Simplest
  Switch1 : Switch  Criteria=u2 > Threshold
  TONV_VariableTimeDebounce : Subsystem  TreatAsAtomicUnit=on  RTWFcnName=TONV_VariableTimeDebounce  RTWFileName=SrvLib
  BTMR_bHtgPlausErrDet : Outport
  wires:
  BSPR_tClntDsT/1 -> Add/1, MinMax1/1
  BSPR_tClntDsStrtHtg/1 -> Add/2
  BSPR_tClntUsT/1 -> MinMax1/2, Add1/1
  BSPR_tClntUsStrtHtg/1 -> Add1/2
  Add/1 -> MinMax/1
  Add1/1 -> MinMax/2
  MinMax/1 -> Relational Operator/1
  Constant4/1 -> TONV_VariableTimeDebounce/3(dT)
  Constant5/1 -> TONV_VariableTimeDebounce/2(T)
  TONV_VariableTimeDebounce/1(y) -> BTMR_bHtgPlausErrDet/1
  COMR_tEnvT/1 -> 2-D Lookup Table2/1
  2-D Lookup Table2/1 -> Relational Operator/2
  MinMax1/1 -> Relational Operator1/1
  Relational Operator/1 -> Logical Operator/1
  Relational Operator1/1 -> Logical Operator/2
  Logical Operator/1 -> TONV_VariableTimeDebounce/1(u)
  Compare To Constant3/1 -> Switch1/2
  Constant1/1 -> Switch1/1
  BMCR_stBmsModeCtrl/1 -> Compare To Constant3/1
  Constant2/1 -> Switch1/3
  Switch1/1 -> Relational Operator1/2

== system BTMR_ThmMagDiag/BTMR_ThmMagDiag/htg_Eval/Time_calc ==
  Enable : EnablePort  StatesWhenEnabling=reset
  Add : Sum
  Constant : Constant  Value=0.1  OutDataTypeStr=uint8
  Constant5 : Constant  Value=BTMR_tiThmHtgEndDiag_C
  Delay : Delay  DelayLength=1  InitialCondition=0
  Logical Operator : Logic  Operator=NOT  Inputs=1  AllPortsSameDT=off  OutDataTypeStr=boolean
  Relational Operator : RelationalOperator  Operator=>  OutDataTypeStr=boolean  RndMeth=Simplest
  BTMR_flgThmHtgTimeEn : Outport
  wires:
  Constant5/1 -> Relational Operator/2
  Relational Operator/1 -> Logical Operator/1
  Logical Operator/1 -> BTMR_flgThmHtgTimeEn/1  "BTMR_flgThmHtgTimeEn"
  Constant/1 -> Add/1
  Delay/1 -> Add/2
  Add/1 -> Delay/1, Relational Operator/1

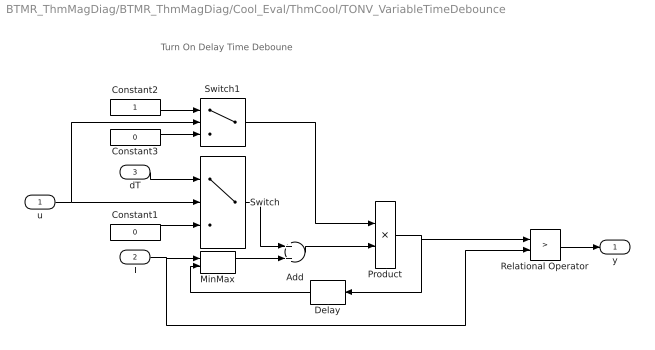
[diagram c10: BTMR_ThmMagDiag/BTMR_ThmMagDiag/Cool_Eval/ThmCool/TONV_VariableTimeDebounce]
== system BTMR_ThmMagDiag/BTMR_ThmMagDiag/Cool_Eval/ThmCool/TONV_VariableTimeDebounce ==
  note: Turn On Delay Time Deboune
  u : Inport
  T : Inport  Port=2
  dT : Inport  Port=3
  Add : Sum
  Constant1 : Constant  Value=0  OutDataTypeStr=single
  Constant2 : Constant  OutDataTypeStr=uint8
  Constant3 : Constant  Value=0  OutDataTypeStr=uint8
  Delay : Delay  DelayLength=1  InitialCondition=0
  MinMax : MinMax  Inputs=2
  Product : Product  OutMin=[0]  OutMax=[65535]  OutDataTypeStr=single
  Relational Operator : RelationalOperator  Operator=>  OutDataTypeStr=boolean  RndMeth=Simplest
  Switch : Switch  Criteria=u2 ~= 0
  Switch1 : Switch  Criteria=u2 ~= 0
  y : Outport
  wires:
  Switch1/1 -> Product/1
  Constant3/1 -> Switch1/3
  Constant2/1 -> Switch1/1
  u/1 -> Switch1/2, Switch/2
  dT/1 -> Switch/1
  Constant1/1 -> Switch/3
  Add/1 -> Product/2
  Product/1 -> Relational Operator/1, Delay/1
  Switch/1 -> Add/1
  Delay/1 -> MinMax/2
  Relational Operator/1 -> y/1
  T/1 -> MinMax/1, Relational Operator/2
  MinMax/1 -> Add/2

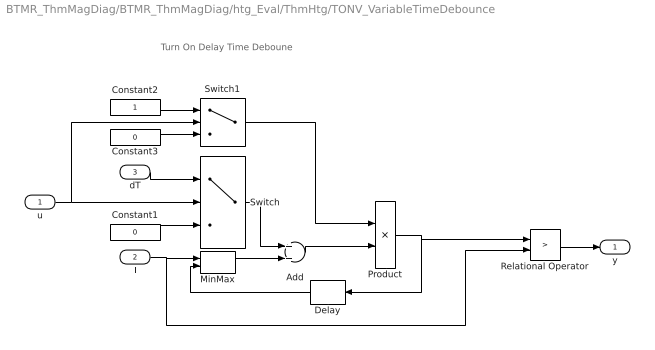
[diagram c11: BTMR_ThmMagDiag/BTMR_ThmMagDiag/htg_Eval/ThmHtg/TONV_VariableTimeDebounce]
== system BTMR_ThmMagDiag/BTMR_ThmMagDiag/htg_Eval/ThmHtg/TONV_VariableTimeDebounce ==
  note: Turn On Delay Time Deboune
  u : Inport
  T : Inport  Port=2
  dT : Inport  Port=3
  Add : Sum
  Constant1 : Constant  Value=0  OutDataTypeStr=single
  Constant2 : Constant  OutDataTypeStr=uint8
  Constant3 : Constant  Value=0  OutDataTypeStr=uint8
  Delay : Delay  DelayLength=1  InitialCondition=0
  MinMax : MinMax  Inputs=2
  Product : Product  OutMin=[0]  OutMax=[65535]  OutDataTypeStr=single
  Relational Operator : RelationalOperator  Operator=>  OutDataTypeStr=boolean  RndMeth=Simplest
  Switch : Switch  Criteria=u2 ~= 0
  Switch1 : Switch  Criteria=u2 ~= 0
  y : Outport
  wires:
  Switch1/1 -> Product/1
  Constant3/1 -> Switch1/3
  Constant2/1 -> Switch1/1
  u/1 -> Switch1/2, Switch/2
  dT/1 -> Switch/1
  Constant1/1 -> Switch/3
  Add/1 -> Product/2
  Product/1 -> Relational Operator/1, Delay/1
  Switch/1 -> Add/1
  Delay/1 -> MinMax/2
  Relational Operator/1 -> y/1
  T/1 -> MinMax/1, Relational Operator/2
  MinMax/1 -> Add/2
